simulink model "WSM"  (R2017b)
settings: Solver=FixedStepDiscrete  StartTime=0.0  StopTime=10.0  FixedStep=0.01  RelTol=1e-3  EnableMultiTasking=on
undefined symbols (not defined in the file): ASWTYPE_FALSE, ASWTYPE_TRUE, CcWSM_KL15WakeupDebTi_ms, CcWSM_ObcWakeupDebTi_ms, Enum_ISPNetWkUpSt, WSM_CONST0_NUMB, WSM_CONST16_NUMB, WSM_CONST1_NUMB, WSM_CONST2_NUMB, WSM_CONST4_NUMB, WSM_CONST64_NUMB, WSM_CONST8_NUMB, WSM_RUNTIME_MS
libraries: AIWAYS_Powertrain_BMS_lib x14

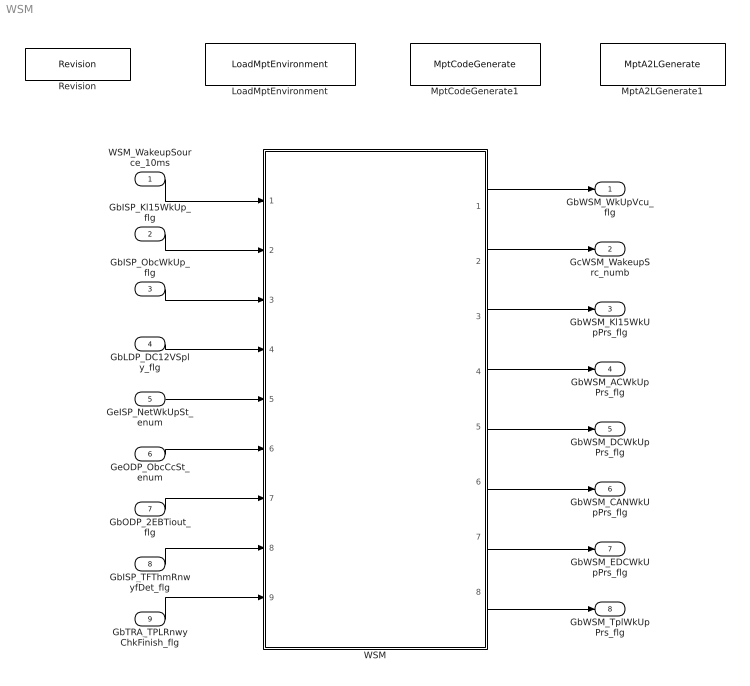
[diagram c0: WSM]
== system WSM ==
  WSM_WakeupSource_10ms : Inport
  GbISP_Kl15WkUp_flg : Inport  Port=2
  GbISP_ObcWkUp_flg : Inport  Port=3
  GbLDP_DC12VSply_flg : Inport  Port=4
  GeISP_NetWkUpSt_enum : Inport  Port=5
  GeODP_ObcCcSt_enum : Inport  Port=6
  GbODP_2EBTiout_flg : Inport  Port=7
  GbISP_TFThmRnwyfDet_flg : Inport  Port=8
  GbTRA_TPLRnwyChkFinish_flg : Inport  Port=9
  LoadMptEnvironment : AIWAYS_Powertrain_BMS_lib/Config/LoadMptEnvironment  ProjectName=Comm  SuppierID=NewPlatformUAES
  MptA2LGenerate1 : AIWAYS_Powertrain_BMS_lib/Config/MptA2LGenerate  SystemSampleTime=-1
  MptCodeGenerate1 : AIWAYS_Powertrain_BMS_lib/Config/MptCodeGenerate  SystemSampleTime=-1
  Revision : AIWAYS_Powertrain_BMS_lib/Config/Revision  curVersion='M105C102'  newVersion='M105C102'
  WSM : Subsystem
  GbWSM_WkUpVcu_flg : Outport
  GcWSM_WakeupSrc_numb : Outport  Port=2
  GbWSM_Kl15WkUpPrs_flg : Outport  Port=3
  GbWSM_ACWkUpPrs_flg : Outport  Port=4
  GbWSM_DCWkUpPrs_flg : Outport  Port=5
  GbWSM_CANWkUpPrs_flg : Outport  Port=6
  GbWSM_EDCWkUpPrs_flg : Outport  Port=7
  GbWSM_TplWkUpPrs_flg : Outport  Port=8
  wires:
  WSM_WakeupSource_10ms/1 -> WSM/1(WSM_WakeupSource_10ms)
  GbISP_Kl15WkUp_flg/1 -> WSM/2(GbISP_Kl15WkUp_flg)
  GbISP_ObcWkUp_flg/1 -> WSM/3(GbISP_ObcWkUp_flg)
  GbLDP_DC12VSply_flg/1 -> WSM/4(GbLDP_DC12VSply_flg)
  GeISP_NetWkUpSt_enum/1 -> WSM/5(GeISP_NetWkUpSt_enum)
  GeODP_ObcCcSt_enum/1 -> WSM/6(GeODP_ObcCcSt_enum)
  GbODP_2EBTiout_flg/1 -> WSM/7(GbODP_2EBTiout_flg)
  WSM/1(GbWSM_WkUpVcu_flg) -> GbWSM_WkUpVcu_flg/1
  WSM/2(GcWSM_WakeupSrc_numb) -> GcWSM_WakeupSrc_numb/1
  WSM/7(GbWSM_EDCWkUpPrs_flg) -> GbWSM_EDCWkUpPrs_flg/1
  WSM/6(GbWSM_CANWkUpPrs_flg) -> GbWSM_CANWkUpPrs_flg/1
  WSM/5(GbWSM_DCWkUpPrs_flg) -> GbWSM_DCWkUpPrs_flg/1
  WSM/4(GbWSM_ACWkUpPrs_flg) -> GbWSM_ACWkUpPrs_flg/1
  WSM/3(GbWSM_Kl15WkUpPrs_flg) -> GbWSM_Kl15WkUpPrs_flg/1
  GbISP_TFThmRnwyfDet_flg/1 -> WSM/8(GbISP_TFThmRnwyfDet_flg)
  GbTRA_TPLRnwyChkFinish_flg/1 -> WSM/9(GbTRA_TPLRnwyChkFinish_flg)
  WSM/8(GbWSM_TplWkUpPrs_flg) -> GbWSM_TplWkUpPrs_flg/1

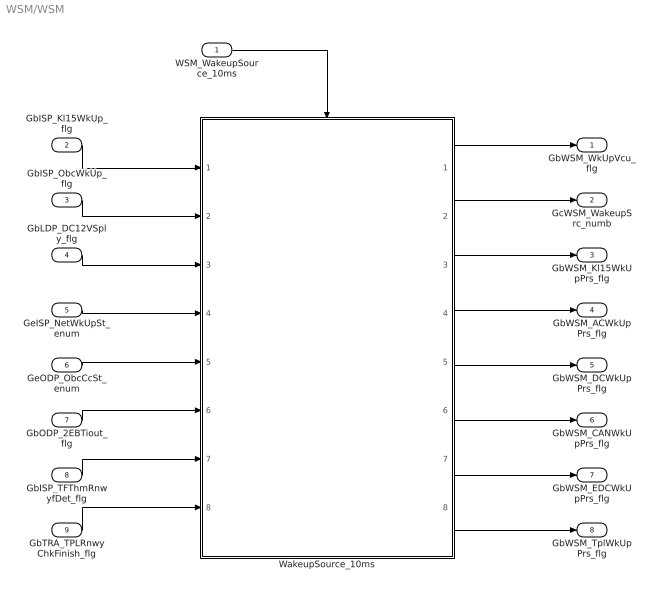
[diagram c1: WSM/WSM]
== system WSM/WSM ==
  WSM_WakeupSource_10ms : Inport
  GbISP_Kl15WkUp_flg : Inport  Port=2
  GbISP_ObcWkUp_flg : Inport  Port=3
  GbLDP_DC12VSply_flg : Inport  Port=4
  GeISP_NetWkUpSt_enum : Inport  Port=5
  GeODP_ObcCcSt_enum : Inport  Port=6
  GbODP_2EBTiout_flg : Inport  Port=7
  GbISP_TFThmRnwyfDet_flg : Inport  Port=8
  GbTRA_TPLRnwyChkFinish_flg : Inport  Port=9
  WakeupSource_10ms : Subsystem
  GbWSM_WkUpVcu_flg : Outport
  GcWSM_WakeupSrc_numb : Outport  Port=2
  GbWSM_Kl15WkUpPrs_flg : Outport  Port=3
  GbWSM_ACWkUpPrs_flg : Outport  Port=4
  GbWSM_DCWkUpPrs_flg : Outport  Port=5
  GbWSM_CANWkUpPrs_flg : Outport  Port=6
  GbWSM_EDCWkUpPrs_flg : Outport  Port=7
  GbWSM_TplWkUpPrs_flg : Outport  Port=8
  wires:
  WSM_WakeupSource_10ms/1 -> WakeupSource_10ms/Trigger
  WakeupSource_10ms/1(GbWSM_WkUpVcu_flg) -> GbWSM_WkUpVcu_flg/1
  WakeupSource_10ms/2(GcWSM_WakeupSrc_numb) -> GcWSM_WakeupSrc_numb/1
  WakeupSource_10ms/3(GbWSM_Kl15WkUpPrs_flg) -> GbWSM_Kl15WkUpPrs_flg/1
  WakeupSource_10ms/4(GbWSM_ACWkUpPrs_flg) -> GbWSM_ACWkUpPrs_flg/1
  WakeupSource_10ms/5(GbWSM_DCWkUpPrs_flg) -> GbWSM_DCWkUpPrs_flg/1
  WakeupSource_10ms/6(GbWSM_CANWkUpPrs_flg) -> GbWSM_CANWkUpPrs_flg/1
  WakeupSource_10ms/7(GbWSM_EDCWkUpPrs_flg) -> GbWSM_EDCWkUpPrs_flg/1
  GbISP_Kl15WkUp_flg/1 -> WakeupSource_10ms/1(GbISP_Kl15WkUp_flg)
  GbISP_ObcWkUp_flg/1 -> WakeupSource_10ms/2(GbISP_ObcWkUp_flg)
  GbLDP_DC12VSply_flg/1 -> WakeupSource_10ms/3(GbLDP_DC12VSply_flg)
  GeISP_NetWkUpSt_enum/1 -> WakeupSource_10ms/4(GeISP_NetWkUpSt_enum)
  GeODP_ObcCcSt_enum/1 -> WakeupSource_10ms/5(GeODP_ObcCcSt_enum)
  GbODP_2EBTiout_flg/1 -> WakeupSource_10ms/6(GbODP_2EBTiout_flg)
  GbISP_TFThmRnwyfDet_flg/1 -> WakeupSource_10ms/7(GbISP_TFThmRnwyfDet_flg)
  GbTRA_TPLRnwyChkFinish_flg/1 -> WakeupSource_10ms/8(GbTRA_TPLRnwyChkFinish_flg)
  WakeupSource_10ms/8(GbWSM_TplWkUpPrs_flg) -> GbWSM_TplWkUpPrs_flg/1

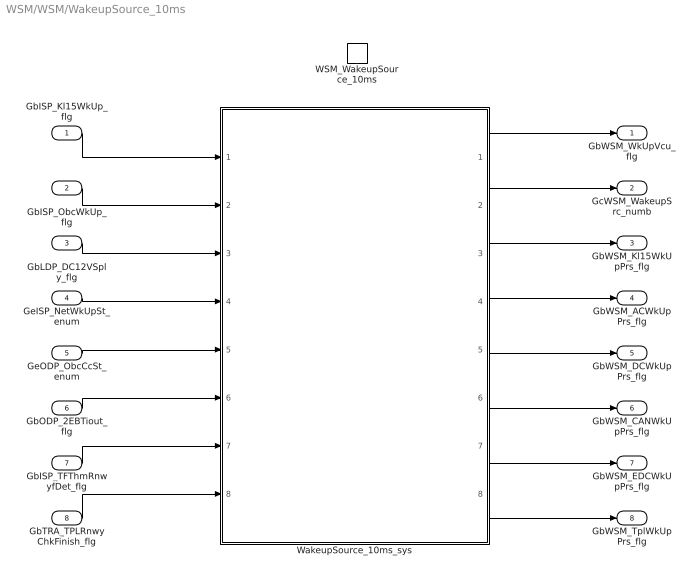
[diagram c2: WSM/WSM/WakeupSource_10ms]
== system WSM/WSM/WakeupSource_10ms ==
  GbISP_Kl15WkUp_flg : Inport
  GbISP_ObcWkUp_flg : Inport  Port=2
  GbLDP_DC12VSply_flg : Inport  Port=3
  GeISP_NetWkUpSt_enum : Inport  Port=4
  GeODP_ObcCcSt_enum : Inport  Port=5
  GbODP_2EBTiout_flg : Inport  Port=6
  GbISP_TFThmRnwyfDet_flg : Inport  Port=7
  GbTRA_TPLRnwyChkFinish_flg : Inport  Port=8
  WSM_WakeupSource_10ms : TriggerPort  TriggerType=function-call  VariantControl=(inherit)
  WakeupSource_10ms_sys : Subsystem
  GbWSM_WkUpVcu_flg : Outport
  GcWSM_WakeupSrc_numb : Outport  Port=2
  GbWSM_Kl15WkUpPrs_flg : Outport  Port=3
  GbWSM_ACWkUpPrs_flg : Outport  Port=4
  GbWSM_DCWkUpPrs_flg : Outport  Port=5
  GbWSM_CANWkUpPrs_flg : Outport  Port=6
  GbWSM_EDCWkUpPrs_flg : Outport  Port=7
  GbWSM_TplWkUpPrs_flg : Outport  Port=8
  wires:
  WakeupSource_10ms_sys/1(GbWSM_WkUpVcu_flg) -> GbWSM_WkUpVcu_flg/1
  WakeupSource_10ms_sys/2(GcWSM_WakeupSrc_numb) -> GcWSM_WakeupSrc_numb/1
  WakeupSource_10ms_sys/3(GbWSM_Kl15WkUpPrs_flg) -> GbWSM_Kl15WkUpPrs_flg/1
  WakeupSource_10ms_sys/4(GbWSM_ACWkUpPrs_flg) -> GbWSM_ACWkUpPrs_flg/1
  WakeupSource_10ms_sys/5(GbWSM_DCWkUpPrs_flg) -> GbWSM_DCWkUpPrs_flg/1
  WakeupSource_10ms_sys/6(GbWSM_CANWkUpPrs_flg) -> GbWSM_CANWkUpPrs_flg/1
  WakeupSource_10ms_sys/7(GbWSM_EDCWkUpPrs_flg) -> GbWSM_EDCWkUpPrs_flg/1
  GbISP_Kl15WkUp_flg/1 -> WakeupSource_10ms_sys/1(GbISP_Kl15WkUp_flg)
  GbISP_ObcWkUp_flg/1 -> WakeupSource_10ms_sys/2(GbISP_ObcWkUp_flg)
  GbLDP_DC12VSply_flg/1 -> WakeupSource_10ms_sys/3(GbLDP_DC12VSply_flg)
  GeISP_NetWkUpSt_enum/1 -> WakeupSource_10ms_sys/4(GeISP_NetWkUpSt_enum)
  GeODP_ObcCcSt_enum/1 -> WakeupSource_10ms_sys/5(GeODP_ObcCcSt_enum)
  GbODP_2EBTiout_flg/1 -> WakeupSource_10ms_sys/6(GbODP_2EBTiout_flg)
  GbISP_TFThmRnwyfDet_flg/1 -> WakeupSource_10ms_sys/7(GbISP_TFThmRnwyfDet_flg)
  GbTRA_TPLRnwyChkFinish_flg/1 -> WakeupSource_10ms_sys/8(GbTRA_TPLRnwyChkFinish_flg)
  WakeupSource_10ms_sys/8(GbWSM_TplWkUpPrs_flg) -> GbWSM_TplWkUpPrs_flg/1

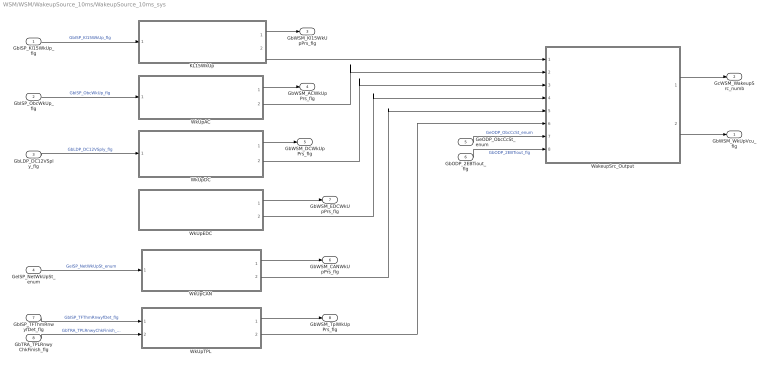
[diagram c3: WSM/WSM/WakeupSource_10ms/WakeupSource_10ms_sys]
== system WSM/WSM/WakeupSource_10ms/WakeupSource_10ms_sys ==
  GbISP_Kl15WkUp_flg : Inport
  GbISP_ObcWkUp_flg : Inport  Port=2
  GbLDP_DC12VSply_flg : Inport  Port=3
  GeISP_NetWkUpSt_enum : Inport  Port=4
  GeODP_ObcCcSt_enum : Inport  Port=5
  GbODP_2EBTiout_flg : Inport  Port=6
  GbISP_TFThmRnwyfDet_flg : Inport  Port=7
  GbTRA_TPLRnwyChkFinish_flg : Inport  Port=8
  KL15WkUp : Subsystem
  WakeupSrc_Output : Subsystem
  WkUpAC : Subsystem
  WkUpCAN : Subsystem
  WkUpDC : Subsystem
  WkUpEDC : Subsystem
  WkUpTPL : Subsystem
  GbWSM_WkUpVcu_flg : Outport
  GcWSM_WakeupSrc_numb : Outport  Port=2
  GbWSM_Kl15WkUpPrs_flg : Outport  Port=3
  GbWSM_ACWkUpPrs_flg : Outport  Port=4
  GbWSM_DCWkUpPrs_flg : Outport  Port=5
  GbWSM_CANWkUpPrs_flg : Outport  Port=6
  GbWSM_EDCWkUpPrs_flg : Outport  Port=7
  GbWSM_TplWkUpPrs_flg : Outport  Port=8
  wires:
  WkUpAC/1(GbWSM_ACWkUpPrs_flg) -> GbWSM_ACWkUpPrs_flg/1
  GbISP_ObcWkUp_flg/1 -> WkUpAC/1(GbISP_ObcWkUp_flg)  "GbISP_ObcWkUp_flg"
  WkUpDC/1(GbWSM_DCWkUpPrs_flg) -> GbWSM_DCWkUpPrs_flg/1
  WkUpCAN/1(GbWSM_CANWkUpPrs_flg) -> GbWSM_CANWkUpPrs_flg/1
  KL15WkUp/1(GbWSM_Kl15WkUpPrs_flg) -> GbWSM_Kl15WkUpPrs_flg/1
  GeISP_NetWkUpSt_enum/1 -> WkUpCAN/1(GeISP_NetWkUpSt_enum)  "GeISP_NetWkUpSt_enum"
  WkUpEDC/1(GbWSM_EDCWkUpPrs_flg) -> GbWSM_EDCWkUpPrs_flg/1
  GbLDP_DC12VSply_flg/1 -> WkUpDC/1(GbLDP_DC12VSply_flg)  "GbLDP_DC12VSply_flg"
  GbISP_Kl15WkUp_flg/1 -> KL15WkUp/1(GbISP_Kl15WkUp_flg)  "GbISP_Kl15WkUp_flg"
  WakeupSrc_Output/1(GcWSM_WakeupSrc_numb) -> GcWSM_WakeupSrc_numb/1
  KL15WkUp/2(LbWSM_Kl15WkUpPrs_flg) -> WakeupSrc_Output/1(LbWSM_Kl15WkUpPrs_flg)
  WkUpAC/2(LbWSM_ACWkUpPrs_flg) -> WakeupSrc_Output/2(LbWSM_ACWkUpPrs_flg)
  WkUpDC/2(LbWSM_DCWkUpPrs_flg) -> WakeupSrc_Output/3(LbWSM_DCWkUpPrs_flg)
  WkUpEDC/2(LbWSM_EDCWkUpPrs_flg) -> WakeupSrc_Output/4(LbWSM_EDCWkUpPrs_flg)
  WkUpCAN/2(LbWSM_CANWkUpPrs_flg) -> WakeupSrc_Output/5(LbWSM_CANWkUpPrs_flg)
  GeODP_ObcCcSt_enum/1 -> WakeupSrc_Output/7(GeODP_ObcCcSt_enum)  "GeODP_ObcCcSt_enum"
  GbODP_2EBTiout_flg/1 -> WakeupSrc_Output/8(GbODP_2EBTiout_flg)  "GbODP_2EBTiout_flg"
  WakeupSrc_Output/2(GbWSM_WkUpVcu_flg) -> GbWSM_WkUpVcu_flg/1
  GbISP_TFThmRnwyfDet_flg/1 -> WkUpTPL/1(GbISP_TFThmRnwyfDet_flg)  "GbISP_TFThmRnwyfDet_flg"
  GbTRA_TPLRnwyChkFinish_flg/1 -> WkUpTPL/2(GbTRA_TPLRnwyChkFinish_flg)  "GbTRA_TPLRnwyChkFinish_flg"
  WkUpTPL/1(GbWSM_TplWkUpPrs_flg) -> GbWSM_TplWkUpPrs_flg/1
  WkUpTPL/2(LbWSM_TplWkUpPrs_flg) -> WakeupSrc_Output/6(LbWSM_TplWkUpPrs_flg)

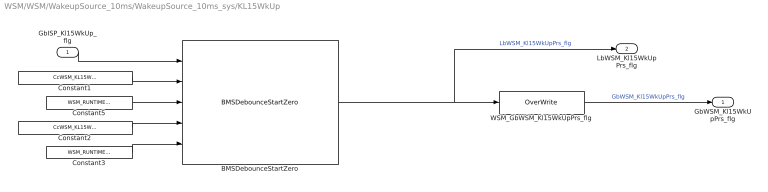
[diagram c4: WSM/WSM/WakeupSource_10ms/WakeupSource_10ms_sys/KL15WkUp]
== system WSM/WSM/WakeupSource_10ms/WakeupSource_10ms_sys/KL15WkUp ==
  GbISP_Kl15WkUp_flg : Inport
  BMSDebounceStartZero : AIWAYS_Powertrain_BMS_lib/Debounce & Delay/BMSDebounceStartZero
  Constant1 : Constant  Value=CcWSM_KL15WakeupDebTi_ms
  Constant2 : Constant  Value=CcWSM_KL15WakeupDebTi_ms
  Constant3 : Constant  Value=WSM_RUNTIME_MS
  Constant5 : Constant  Value=WSM_RUNTIME_MS
  WSM_GbWSM_Kl15WkUpPrs_flg : AIWAYS_Powertrain_BMS_lib/Signals/OverWrite  OverWrite_Value=CbWSM_Kl15WkUpPrsOvr_flg  OverWrite_flag=CbWSM_Kl15WkUpPrsOvrSwt_flg
  GbWSM_Kl15WkUpPrs_flg : Outport
  LbWSM_Kl15WkUpPrs_flg : Outport  Port=2
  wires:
  WSM_GbWSM_Kl15WkUpPrs_flg/1 -> GbWSM_Kl15WkUpPrs_flg/1  "GbWSM_Kl15WkUpPrs_flg"
  Constant2/1 -> BMSDebounceStartZero/4
  Constant1/1 -> BMSDebounceStartZero/2
  Constant5/1 -> BMSDebounceStartZero/3
  BMSDebounceStartZero/1 -> LbWSM_Kl15WkUpPrs_flg/1, WSM_GbWSM_Kl15WkUpPrs_flg/1  "LbWSM_Kl15WkUpPrs_flg"
  GbISP_Kl15WkUp_flg/1 -> BMSDebounceStartZero/1
  Constant3/1 -> BMSDebounceStartZero/5

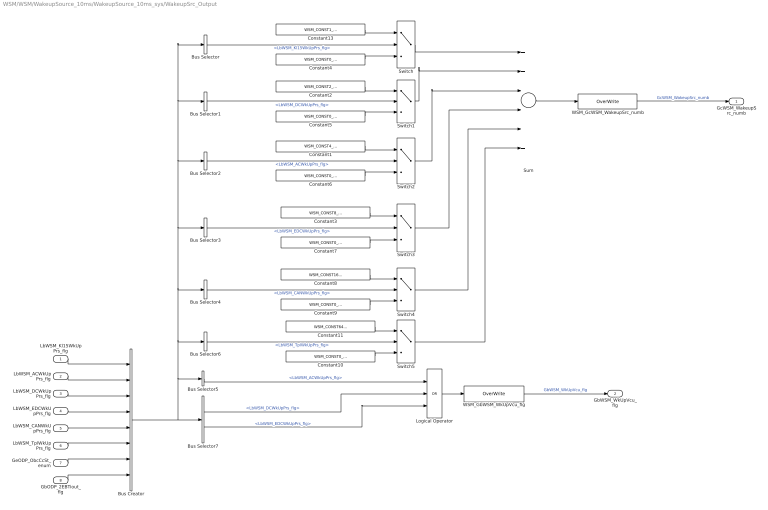
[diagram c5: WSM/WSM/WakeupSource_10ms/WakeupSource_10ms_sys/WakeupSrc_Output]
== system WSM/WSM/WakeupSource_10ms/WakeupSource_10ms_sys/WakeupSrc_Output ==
  LbWSM_Kl15WkUpPrs_flg : Inport
  LbWSM_ACWkUpPrs_flg : Inport  Port=2
  LbWSM_DCWkUpPrs_flg : Inport  Port=3
  LbWSM_EDCWkUpPrs_flg : Inport  Port=4
  LbWSM_CANWkUpPrs_flg : Inport  Port=5
  LbWSM_TplWkUpPrs_flg : Inport  Port=6
  GeODP_ObcCcSt_enum : Inport  Port=7
  GbODP_2EBTiout_flg : Inport  Port=8
  Bus Creator : BusCreator  Inputs=8
  Bus Selector : BusSelector  OutputSignals=LbWSM_Kl15WkUpPrs_flg
  Bus Selector1 : BusSelector  OutputSignals=LbWSM_DCWkUpPrs_flg
  Bus Selector2 : BusSelector  OutputSignals=LbWSM_ACWkUpPrs_flg
  Bus Selector3 : BusSelector  OutputSignals=LbWSM_EDCWkUpPrs_flg
  Bus Selector4 : BusSelector  OutputSignals=LbWSM_CANWkUpPrs_flg
  Bus Selector5 : BusSelector  OutputSignals=LbWSM_ACWkUpPrs_flg
  Bus Selector6 : BusSelector  OutputSignals=LbWSM_TplWkUpPrs_flg
  Bus Selector7 : BusSelector  OutputSignals=LbWSM_DCWkUpPrs_flg,LbWSM_EDCWkUpPrs_flg
  Constant1 : Constant  Value=WSM_CONST4_NUMB
  Constant{4..7,9..10} (6 alike) : Constant  Value=WSM_CONST0_NUMB
  Constant11 : Constant  Value=WSM_CONST64_NUMB
  Constant13 : Constant  Value=WSM_CONST1_NUMB
  Constant2 : Constant  Value=WSM_CONST2_NUMB
  Constant3 : Constant  Value=WSM_CONST8_NUMB
  Constant8 : Constant  Value=WSM_CONST16_NUMB
  Logical Operator : Logic  Operator=OR  Inputs=3  AllPortsSameDT=off  OutDataTypeStr=boolean
  Sum : Sum  Inputs=++++++  OutDataTypeStr=Inherit: Inherit via back propagation  RndMeth=Zero
  Switch{,1..5} (6 alike) : Switch  Criteria=u2 ~= 0
  WSM_GbWSM_WkUpVcu_flg : AIWAYS_Powertrain_BMS_lib/Signals/OverWrite  OverWrite_Value=CbWSM_WkUpVcuOvr_flg  OverWrite_flag=CbWSM_WkUpVcuOvrSwt_flg
  WSM_GcWSM_WakeupSrc_numb : AIWAYS_Powertrain_BMS_lib/Signals/OverWrite  OverWrite_Value=CcWSM_WakeupSrcOvr_numb  OverWrite_flag=CbWSM_WakeupSrcOvrSwt_flg
  GcWSM_WakeupSrc_numb : Outport
  GbWSM_WkUpVcu_flg : Outport  Port=2
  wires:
  Constant13/1 -> Switch/1
  Constant3/1 -> Switch3/1
  Switch/1 -> Sum/1
  Sum/1 -> WSM_GcWSM_WakeupSrc_numb/1
  Constant4/1 -> Switch/3
  Constant5/1 -> Switch1/3
  Constant6/1 -> Switch2/3
  Constant7/1 -> Switch3/3
  WSM_GcWSM_WakeupSrc_numb/1 -> GcWSM_WakeupSrc_numb/1  "GcWSM_WakeupSrc_numb"
  Constant1/1 -> Switch2/1
  Constant2/1 -> Switch1/1
  Constant9/1 -> Switch4/3
  Constant8/1 -> Switch4/1
  Switch1/1 -> Sum/2
  Switch2/1 -> Sum/3
  Switch3/1 -> Sum/4
  Switch4/1 -> Sum/5
  WSM_GbWSM_WkUpVcu_flg/1 -> GbWSM_WkUpVcu_flg/1  "GbWSM_WkUpVcu_flg"
  LbWSM_Kl15WkUpPrs_flg/1 -> Bus Creator/1
  LbWSM_ACWkUpPrs_flg/1 -> Bus Creator/2
  LbWSM_DCWkUpPrs_flg/1 -> Bus Creator/3
  LbWSM_EDCWkUpPrs_flg/1 -> Bus Creator/4
  LbWSM_CANWkUpPrs_flg/1 -> Bus Creator/5
  Bus Selector/1 -> Switch/2  "<LbWSM_Kl15WkUpPrs_flg>"
  Bus Selector1/1 -> Switch1/2  "<LbWSM_DCWkUpPrs_flg>"
  Bus Selector2/1 -> Switch2/2  "<LbWSM_ACWkUpPrs_flg>"
  Bus Selector3/1 -> Switch3/2  "<LbWSM_EDCWkUpPrs_flg>"
  Bus Selector4/1 -> Switch4/2  "<LbWSM_CANWkUpPrs_flg>"
  Logical Operator/1 -> WSM_GbWSM_WkUpVcu_flg/1
  Bus Selector5/1 -> Logical Operator/1  "<LbWSM_ACWkUpPrs_flg>"
  Bus Selector7/1 -> Logical Operator/2  "<LbWSM_DCWkUpPrs_flg>"
  Bus Selector7/2 -> Logical Operator/3  "<LbWSM_EDCWkUpPrs_flg>"
  Bus Creator/1 -> Bus Selector6/1, Bus Selector/1, Bus Selector1/1, Bus Selector2/1, Bus Selector3/1, Bus Selector4/1, Bus Selector5/1, Bus Selector7/1
  LbWSM_TplWkUpPrs_flg/1 -> Bus Creator/6
  GeODP_ObcCcSt_enum/1 -> Bus Creator/7
  GbODP_2EBTiout_flg/1 -> Bus Creator/8
  Bus Selector6/1 -> Switch5/2  "<LbWSM_TplWkUpPrs_flg>"
  Constant10/1 -> Switch5/3
  Constant11/1 -> Switch5/1
  Switch5/1 -> Sum/6

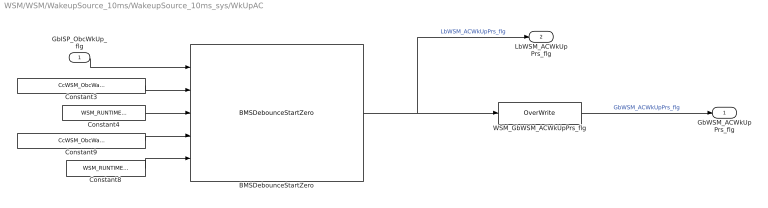
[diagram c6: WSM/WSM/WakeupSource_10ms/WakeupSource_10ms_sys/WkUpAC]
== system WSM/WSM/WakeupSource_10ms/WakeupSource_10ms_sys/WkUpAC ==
  GbISP_ObcWkUp_flg : Inport
  BMSDebounceStartZero : AIWAYS_Powertrain_BMS_lib/Debounce & Delay/BMSDebounceStartZero
  Constant3 : Constant  Value=CcWSM_ObcWakeupDebTi_ms
  Constant4 : Constant  Value=WSM_RUNTIME_MS
  Constant8 : Constant  Value=WSM_RUNTIME_MS
  Constant9 : Constant  Value=CcWSM_ObcWakeupDebTi_ms
  WSM_GbWSM_ACWkUpPrs_flg : AIWAYS_Powertrain_BMS_lib/Signals/OverWrite  OverWrite_Value=CbWSM_ACWkUpPrsOvr_flg  OverWrite_flag=CbWSM_ACWkUpPrsOvrSwt_flg
  GbWSM_ACWkUpPrs_flg : Outport
  LbWSM_ACWkUpPrs_flg : Outport  Port=2
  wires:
  WSM_GbWSM_ACWkUpPrs_flg/1 -> GbWSM_ACWkUpPrs_flg/1  "GbWSM_ACWkUpPrs_flg"
  Constant9/1 -> BMSDebounceStartZero/4
  Constant8/1 -> BMSDebounceStartZero/5
  Constant3/1 -> BMSDebounceStartZero/2
  Constant4/1 -> BMSDebounceStartZero/3
  GbISP_ObcWkUp_flg/1 -> BMSDebounceStartZero/1
  BMSDebounceStartZero/1 -> LbWSM_ACWkUpPrs_flg/1, WSM_GbWSM_ACWkUpPrs_flg/1  "LbWSM_ACWkUpPrs_flg"

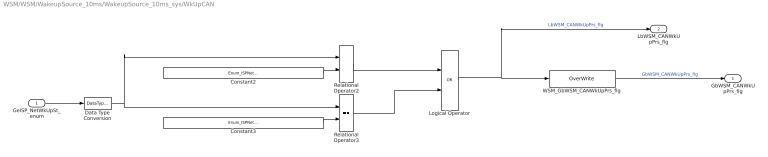
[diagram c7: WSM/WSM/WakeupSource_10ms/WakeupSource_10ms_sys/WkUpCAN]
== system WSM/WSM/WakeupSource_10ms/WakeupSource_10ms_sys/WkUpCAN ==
  GeISP_NetWkUpSt_enum : Inport
  Constant2 : Constant  Value=Enum_ISPNetWkUpSt.Enum_ISPNetWkUpSt_NormalOperation
  Constant3 : Constant  Value=Enum_ISPNetWkUpSt.Enum_ISPNetWkUpSt_RepeatMessage
  Data Type Conversion : DataTypeConversion
  Logical Operator : Logic  Operator=OR  AllPortsSameDT=off  OutDataTypeStr=boolean
  Relational Operator2 : RelationalOperator  Operator===  OutDataTypeStr=boolean
  Relational Operator3 : RelationalOperator  Operator===  OutDataTypeStr=boolean
  WSM_GbWSM_CANWkUpPrs_flg : AIWAYS_Powertrain_BMS_lib/Signals/OverWrite  OverWrite_Value=CbWSM_CANWkUpPrsOvr_flg  OverWrite_flag=CbWSM_CANWkUpPrsOvrSwt_flg
  GbWSM_CANWkUpPrs_flg : Outport
  LbWSM_CANWkUpPrs_flg : Outport  Port=2
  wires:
  WSM_GbWSM_CANWkUpPrs_flg/1 -> GbWSM_CANWkUpPrs_flg/1  "GbWSM_CANWkUpPrs_flg"
  Constant2/1 -> Relational Operator2/2
  GeISP_NetWkUpSt_enum/1 -> Data Type Conversion/1
  Data Type Conversion/1 -> Relational Operator2/1, Relational Operator3/1
  Constant3/1 -> Relational Operator3/2
  Logical Operator/1 -> WSM_GbWSM_CANWkUpPrs_flg/1, LbWSM_CANWkUpPrs_flg/1  "LbWSM_CANWkUpPrs_flg"
  Relational Operator2/1 -> Logical Operator/1
  Relational Operator3/1 -> Logical Operator/2

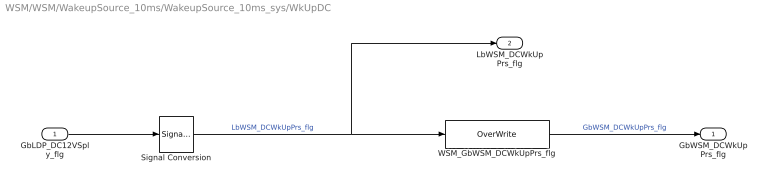
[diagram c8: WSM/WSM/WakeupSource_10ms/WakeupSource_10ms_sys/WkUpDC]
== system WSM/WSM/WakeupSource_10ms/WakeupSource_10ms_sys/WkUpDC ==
  GbLDP_DC12VSply_flg : Inport
  Signal Conversion : SignalConversion  ConversionOutput=Contiguous copy  OverrideOpt=off
  WSM_GbWSM_DCWkUpPrs_flg : AIWAYS_Powertrain_BMS_lib/Signals/OverWrite  OverWrite_Value=CbWSM_DCWkUpPrsOvr_flg  OverWrite_flag=CbWSM_DCWkUpPrsOvrSwt_flg
  GbWSM_DCWkUpPrs_flg : Outport
  LbWSM_DCWkUpPrs_flg : Outport  Port=2
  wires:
  WSM_GbWSM_DCWkUpPrs_flg/1 -> GbWSM_DCWkUpPrs_flg/1  "GbWSM_DCWkUpPrs_flg"
  GbLDP_DC12VSply_flg/1 -> Signal Conversion/1
  Signal Conversion/1 -> LbWSM_DCWkUpPrs_flg/1, WSM_GbWSM_DCWkUpPrs_flg/1  "LbWSM_DCWkUpPrs_flg"

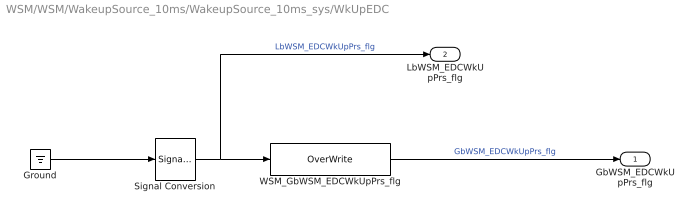
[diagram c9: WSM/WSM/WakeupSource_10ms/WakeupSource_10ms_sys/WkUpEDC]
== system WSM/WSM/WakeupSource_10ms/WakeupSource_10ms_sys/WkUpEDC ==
  Ground : Ground
  Signal Conversion : SignalConversion  ConversionOutput=Contiguous copy  OverrideOpt=off
  WSM_GbWSM_EDCWkUpPrs_flg : AIWAYS_Powertrain_BMS_lib/Signals/OverWrite  OverWrite_Value=CbWSM_EDCWkUpPrsOvr_flg  OverWrite_flag=CbWSM_EDCWkUpPrsOvrSwt_flg
  GbWSM_EDCWkUpPrs_flg : Outport
  LbWSM_EDCWkUpPrs_flg : Outport  Port=2
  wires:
  WSM_GbWSM_EDCWkUpPrs_flg/1 -> GbWSM_EDCWkUpPrs_flg/1  "GbWSM_EDCWkUpPrs_flg"
  Signal Conversion/1 -> LbWSM_EDCWkUpPrs_flg/1, WSM_GbWSM_EDCWkUpPrs_flg/1  "LbWSM_EDCWkUpPrs_flg"
  Ground/1 -> Signal Conversion/1

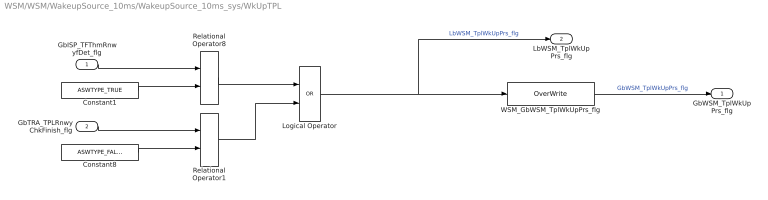
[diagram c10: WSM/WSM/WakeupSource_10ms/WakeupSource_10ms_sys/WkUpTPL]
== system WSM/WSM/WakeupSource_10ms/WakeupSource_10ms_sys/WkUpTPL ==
  GbISP_TFThmRnwyfDet_flg : Inport
  GbTRA_TPLRnwyChkFinish_flg : Inport  Port=2
  Constant1 : Constant  Value=ASWTYPE_TRUE
  Constant8 : Constant  Value=ASWTYPE_FALSE
  Logical Operator : Logic  Operator=OR  AllPortsSameDT=off  OutDataTypeStr=boolean
  Relational Operator1 : RelationalOperator  Operator===  OutDataTypeStr=boolean
  Relational Operator8 : RelationalOperator  Operator===  OutDataTypeStr=boolean
  WSM_GbWSM_TplWkUpPrs_flg : AIWAYS_Powertrain_BMS_lib/Signals/OverWrite  OverWrite_Value=CbWSM_TplWkUpPrsOvr_flg  OverWrite_flag=CbWSM_TplWkUpPrsOvrSwt_flg
  GbWSM_TplWkUpPrs_flg : Outport
  LbWSM_TplWkUpPrs_flg : Outport  Port=2
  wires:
  GbISP_TFThmRnwyfDet_flg/1 -> Relational Operator8/1
  GbTRA_TPLRnwyChkFinish_flg/1 -> Relational Operator1/1
  Relational Operator8/1 -> Logical Operator/1
  Relational Operator1/1 -> Logical Operator/2
  Logical Operator/1 -> WSM_GbWSM_TplWkUpPrs_flg/1, LbWSM_TplWkUpPrs_flg/1  "LbWSM_TplWkUpPrs_flg"
  WSM_GbWSM_TplWkUpPrs_flg/1 -> GbWSM_TplWkUpPrs_flg/1  "GbWSM_TplWkUpPrs_flg"
  Constant1/1 -> Relational Operator8/2
  Constant8/1 -> Relational Operator1/2
